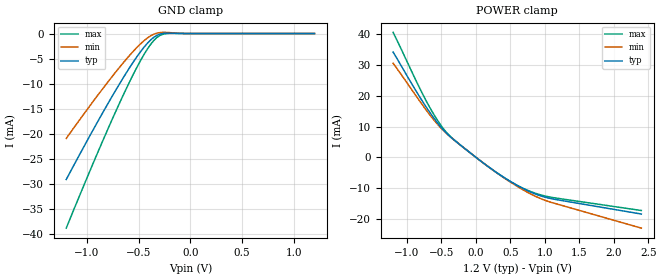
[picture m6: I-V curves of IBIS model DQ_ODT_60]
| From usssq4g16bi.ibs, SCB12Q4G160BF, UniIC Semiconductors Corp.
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|   Model DQ_ODT_60
[Model] DQ_ODT_60
Model_type Input
Polarity   Non-Inverting
Enable   Active-High
Vinl =  8.300E-01
Vinh =  9.700E-01
C_comp   8.081E-13   8.067E-13   8.176E-13
C_comp_power_clamp   2.436E-13   2.328E-13   2.608E-13
C_comp_gnd_clamp   5.645E-13   5.568E-13   5.739E-13
[Model Spec]
Vinh   9.700E-01   9.250E-01   1.015E+00
Vinl   8.300E-01   7.850E-01   8.750E-01
[Temperature Range]   45.000   95.000   -40.000
[Voltage Range]   1.200E+00   1.140E+00   1.260E+00
[C Comp Corner]
C_comp_power_clamp   2.436E-13   2.328E-13   2.608E-13
C_comp_gnd_clamp   5.645E-13   5.739E-13   5.568E-13
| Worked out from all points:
|   GND clamp passes 1 mA (typ) near -0.37 V on its own axis
|   POWER clamp passes 1 mA (typ) near -0.06 V on its own axis
[GND_clamp]
|Voltage   I(typ)   I(min)   I(max)
-1.2V     -29.15mA   -20.95mA   -38.87mA
-875mV    -16.84mA   -11.78mA   -22.78mA
-750mV    -12.33mA   -8.433mA   -16.88mA
-625mV    -8.042mA   -5.268mA   -11.25mA
-525mV    -4.883mA   -2.963mA   -7.072mA
-450mV    -2.787mA   -1.473mA   -4.255mA
-375mV    -1.118mA   -356.8uA   -1.929mA
-325mV    -387.2uA   68.84uA    -829.1uA
-275mV    -25.32uA   224.4uA    -210.6uA
-200mV    74.01uA    182.3uA    31.47uA
-25mV     0A         0A         0A
1.2V      0A         0A         0A
[POWER_clamp]
|Voltage   I(typ)   I(min)   I(max)
-1.2V     34.25mA    30.61mA    40.69mA
-750mV    17.39mA    16.29mA    19.64mA
-625mV    13.27mA    12.6mA     14.54mA
-500mV    9.64mA     9.372mA    10.19mA
-425mV    7.824mA    7.724mA    8.068mA
-325mV    5.812mA    5.789mA    5.89mA
225mV     -3.778mA   -3.801mA   -3.811mA
625mV     -9.493mA   -9.813mA   -9.422mA
800mV     -11.41mA   -12mA      -11.21mA
950mV     -12.64mA   -13.55mA   -12.31mA
1.175V    -13.82mA   -15.22mA   -13.33mA
2.4V      -18.49mA   -23.08mA   -17.34mA
